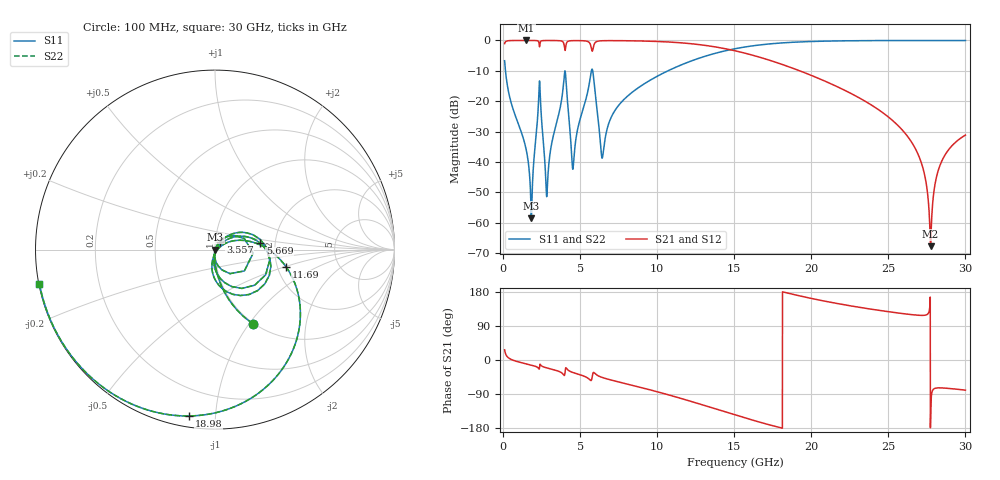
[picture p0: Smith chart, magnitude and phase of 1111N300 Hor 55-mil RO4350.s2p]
# GHz S MA R 50
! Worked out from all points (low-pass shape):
!   3201 points, 100 MHz to 30 GHz, reference 50 ohm
!   highest |S21| = -0.01 dB at 1.511 GHz (marker M1); lowest = -67.7 dB at 27.74 GHz (marker M2)
!   |S21| within 3 dB of the highest: start of sweep to 4.007 GHz; 5.826 GHz to 14.69 GHz (8.865 GHz wide, 86.4 % of centre)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
!   lowest |S11| = -58.6 dB at 1.838 GHz (marker M3), VSWR 1.00, Z = 50.1 - j0.0261 ohm
!   |S11| at or under -10 dB: 156.5 MHz to 5.732 GHz (5.576 GHz wide, 189 % of centre); 5.816 GHz to 10.7 GHz (4.885 GHz wide, 59.1 % of centre)
!   |S22| runs from -58.6 to 0.0 dB; largest |S21 - S12| = 1.5e-10
!   S11 on the Smith chart (normalised r, x): 100 MHz: 0.99, -1.04; 3.557 GHz: 1.06, +0.09; 5.669 GHz: 1.67, +0.13; 11.69 GHz: 2.23, -0.52; 18.98 GHz: 0.06, -0.86; 30 GHz: 0.00, -0.10
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0.1  0.4635 -63.1  0.8859 26.9  0.8859 26.9  0.4635 -63.1
1.510906  0.0155 -97.3  0.9989 -10.3  0.9989 -10.3  0.0155 -97.3
1.837938  0.001177 -12.8  0.9986 -13.6  0.9986 -13.6  0.001177 -12.8
2.333156  0.1525 29.5  0.9018 -24.2  0.9018 -24.2  0.1525 29.5
2.837719  0.002704 -8.7  0.997 -20.9  0.997 -20.9  0.002704 -8.7
3.557187  0.0533 55.7  0.9933 -29.0  0.9933 -29.0  0.0533 55.7
4.033719  0.3087 -34.4  0.6926 -27.1  0.6926 -27.1  0.3087 -34.4
4.547625  0.008132 -5.0  0.9923 -33.2  0.9923 -33.2  0.008132 -5.0
5.089563  0.06076 43.1  0.9905 -40.2  0.9905 -40.2  0.06076 43.1
5.668875  0.2542 8.2  0.8542 -53.7  0.8542 -53.7  0.2542 8.2
6.45375  0.0119 -21.3  0.9885 -46.3  0.9885 -46.3  0.0119 -21.3
7.416156  0.08022 29.7  0.9915 -57.0  0.9915 -57.0  0.08022 29.7
10.06978  0.2627 4.7  0.9599 -84.5  0.9599 -84.5  0.2627 4.7
11.68625  0.4076 -13.7  0.9075 -103.1  0.9075 -103.1  0.4076 -13.7
15.05  0.73 -55.4  0.6757 -145.0  0.6757 -145.0  0.73 -55.4
18.98372  0.9378 -98.8  0.3351 171.7  0.3351 171.7  0.9378 -98.8
20.03956  0.9607 -108.2  0.2634 162.2  0.2634 162.2  0.9607 -108.2
25.01978  0.9954 -143.4  0.05445 127.4  0.05445 127.4  0.9954 -143.4
26.98197  0.9969 -154.2  0.01243 118.0  0.01243 118.0  0.9969 -154.2
27.73881  0.9969 -158.1  0.0004105 -160.0  0.0004105 -160.0  0.9969 -158.1
28.41156  0.9969 -161.5  0.009577 -73.6  0.009577 -73.6  0.9969 -161.5
30  0.9965 -168.9  0.02767 -79.4  0.02767 -79.4  0.9965 -168.9
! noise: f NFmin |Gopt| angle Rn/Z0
0.1  0.0007  0.7471  2.033  0.0005565
3.417  0.01457  0.6191  24.74  0.006819
6.743  0.02903  0.633  47.79  0.01256
10.06  0.02729  0.4934  65.1  0.006888
13.39  0.03884  0.5463  80.66  0.009407
16.7  0.0609  0.6572  97.18  0.01564
20.03  0.1101  0.7901  115.8  0.03163
23.35  0.2564  0.9043  134.9  0.08785
26.67  1.447  0.9821  152.8  1.041
30  0.9606  0.9725  168.8  0.07753
